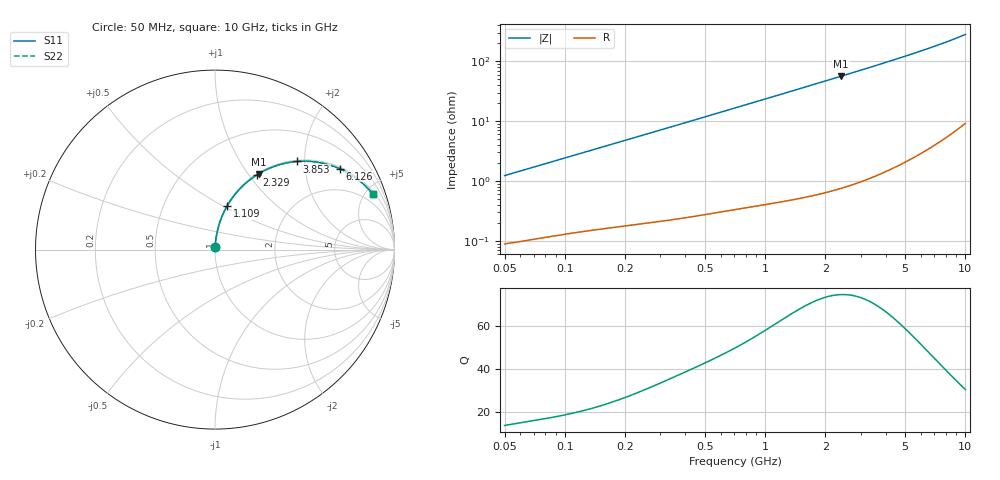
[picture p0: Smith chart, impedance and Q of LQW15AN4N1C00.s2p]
!Murata Part Number: LQW15AN4N1C00
!These Parameters are Measured in Series Mode Connection
!  o--[Z]--o
!Port1  Port2
!  o-------o
!Freq. Start=50[MHz] Stop=10[GHz], 401[Steps]
# Hz S RI R 50
!Freq.(Hz)	S 11(Real)	S 11(Imag)	S 21(Real)	S 21(Imag)	S 12(Real)	S 12(Imag)	S 22(Real)	S 22(Imag)
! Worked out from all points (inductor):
!   401 points, 50 MHz to 10 GHz, reference 50 ohm
!   read as one part in series: L = 3.89 nH near 51.34 MHz
!   highest Q = 74.6 at 2.392 GHz (marker M1), where L = 3.74 nH
!   S11 on the Smith chart (normalised r, x): 50 MHz: 1.00, +0.02; 1.109 GHz: 1.01, +0.52; 2.329 GHz: 1.01, +1.09; 3.853 GHz: 1.03, +1.84; 6.126 GHz: 1.06, +3.04; 10 GHz: 1.18, +5.59
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5e7  0.00104 0.0123  0.999 -0.0123  0.999 -0.0123  0.00104 0.0123
1.214486e8  0.00227 0.0291  0.9977 -0.0291  0.9977 -0.0291  0.00227 0.0291
1.956524e8  0.0039 0.0463  0.9961 -0.0463  0.9961 -0.0463  0.0039 0.0463
2.949953e8  0.0069 0.0691  0.9931 -0.0691  0.9931 -0.0691  0.0069 0.0691
4.689809e8  0.0146 0.1084  0.9854 -0.1084  0.9854 -0.1084  0.0146 0.1084
7.071068e8  0.0298 0.1602  0.9702 -0.1602  0.9702 -0.1602  0.0298 0.1602
8.974936e8  0.0455 0.1996  0.9545 -0.1996  0.9545 -0.1996  0.0455 0.1996
1.10936e9  0.0665 0.241  0.9335 -0.241  0.9335 -0.241  0.0665 0.241
1.389525e9  0.0989 0.2911  0.9011 -0.2911  0.9011 -0.2911  0.0989 0.2911
1.717543e9  0.1424 0.3425  0.8576 -0.3425  0.8576 -0.3425  0.1424 0.3425
2.013439e9  0.1852 0.3817  0.8148 -0.3817  0.8148 -0.3817  0.1852 0.3817
2.329253e9  0.233 0.4161  0.767 -0.4161  0.767 -0.4161  0.233 0.4161
2.391784e9  0.2426 0.422  0.7574 -0.422  0.7574 -0.422  0.2426 0.422
3.076244e9  0.3474 0.4693  0.6526 -0.4693  0.6526 -0.4693  0.3474 0.4693
3.853138e9  0.458 0.4909  0.542 -0.4909  0.542 -0.4909  0.458 0.4909
4.171863e9  0.4993 0.4924  0.5007 -0.4924  0.5007 -0.4924  0.4993 0.4924
5.021877e9  0.5959 0.4823  0.4041 -0.4823  0.4041 -0.4823  0.5959 0.4823
6.125686e9  0.6942 0.4509  0.3058 -0.4509  0.3058 -0.4509  0.6942 0.4509
6.993273e9  0.7535 0.42  0.2465 -0.42  0.2465 -0.42  0.7535 0.42
7.983737e9  0.8061 0.3829  0.1939 -0.3829  0.1939 -0.3829  0.8061 0.3829
9.114482e9  0.8515 0.3413  0.1485 -0.3413  0.1485 -0.3413  0.8515 0.3413
1e10  0.8789 0.3103  0.1211 -0.3103  0.1211 -0.3103  0.8789 0.3103
